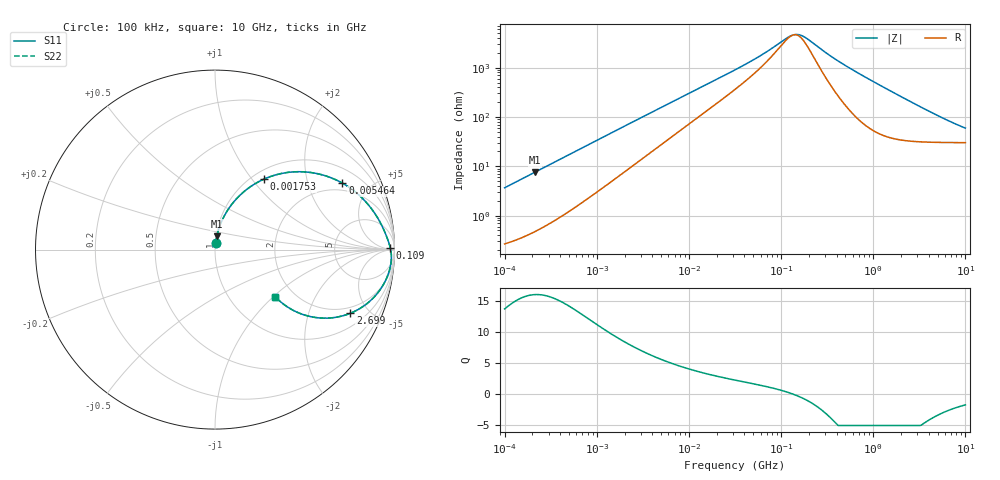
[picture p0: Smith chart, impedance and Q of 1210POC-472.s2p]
# MHz S MA R 50
!Freq  MagS11  AngS11  MagS21  AngS21  MagS12  AngS12  MagS22  AngS22
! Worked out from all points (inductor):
!   801 points, 100 kHz to 10 GHz, reference 50 ohm
!   read as one part in series: L = 5.77 uH near 105.9 kHz
!   highest Q = 16 at 211.3 kHz (marker M1), where L = 5.67 uH
!   self-resonance near 136.6 MHz
!   S11 on the Smith chart (normalised r, x): 100 kHz: 1.01, +0.07; 1.753 MHz: 1.13, +1.14; 5.464 MHz: 1.62, +3.34; 109 MHz: 68, +33; 2.699 GHz: 1.64, -3.80; 10 GHz: 1.60, -1.03
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0.1  0.03656 83.7  0.9967 -2.1  0.9967 -2.1  0.03656 83.7
0.2113489  0.07485 82.1  0.9925 -4.3  0.9925 -4.3  0.07485 82.1
0.6878599  0.2246 72.6  0.9572 -12.9  0.9572 -12.9  0.2246 72.6
1.122018  0.3411 64.8  0.9089 -19.9  0.9089 -19.9  0.3411 64.8
1.752871  0.4763 55.4  0.8278 -28.3  0.8278 -28.3  0.4763 55.4
2.859236  0.6342 43.2  0.6908 -38.9  0.6908 -38.9  0.6342 43.2
4.663908  0.7668 31.1  0.5244 -49.1  0.5244 -49.1  0.7668 31.1
5.463865  0.8003 27.6  0.4709 -51.9  0.4709 -51.9  0.8003 27.6
11.38282  0.8999 14.8  0.2645 -60.5  0.2645 -60.5  0.8999 14.8
31.62278  0.9529 5.6  0.1057 -60.8  0.1057 -60.8  0.9529 5.6
61.30558  0.9681 2.5  0.05365 -52.2  0.05365 -52.2  0.9681 2.5
109.0184  0.9764 0.7  0.02617 -25.4  0.02617 -25.4  0.9764 0.7
131.4468  0.9785 0.1  0.02162 -5.1  0.02162 -5.1  0.9785 0.1
151.7924  0.9798 -0.3  0.02085 14.7  0.02085 14.7  0.9798 -0.3
175.2871  0.981 -0.7  0.02286 33.6  0.02286 33.6  0.981 -0.7
217.5204  0.9825 -1.4  0.0302 53.9  0.0302 53.9  0.9825 -1.4
486.9675  0.9826 -4.9  0.08643 75.9  0.08643 75.9  0.9826 -4.9
1474.857  0.9353 -15.3  0.2657 68.4  0.2657 68.4  0.9353 -15.3
2699.293  0.833 -25.2  0.4319 55.2  0.4319 55.2  0.833 -25.2
4800.097  0.6586 -34.7  0.5927 39.3  0.5927 39.3  0.6586 -34.7
7079.458  0.5266 -38.2  0.6708 29.1  0.6708 29.1  0.5266 -38.2
10000  0.4253 -38.0  0.7146 21.5  0.7146 21.5  0.4253 -38.0
